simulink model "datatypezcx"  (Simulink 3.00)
settings: Solver=FixedStepDiscrete  SolverMode=SingleTasking  StartTime=0.0  StopTime=4  FixedStep=.01  RelTol=1e-3

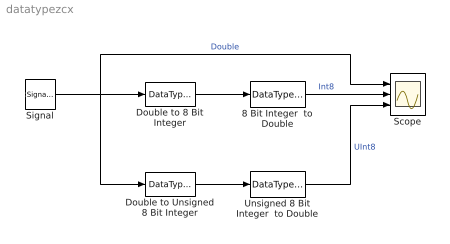
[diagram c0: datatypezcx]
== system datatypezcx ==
  8 Bit Integer  to Double : DataTypeConversion  DataType=double  SaturateOnIntegerOverflow=on
  Double to 8 Bit Integer : DataTypeConversion  DataType=int8  SaturateOnIntegerOverflow=on
  Double to Unsigned 8 Bit Integer : DataTypeConversion  DataType=uint8  SaturateOnIntegerOverflow=on
  Scope : Scope  NumInputPorts=3
  Signal : SignalGenerator  WaveForm=sine  Amplitude=150  Frequency=1  Units=Hertz
  Unsigned 8 Bit Integer  to Double : DataTypeConversion  DataType=double  SaturateOnIntegerOverflow=on
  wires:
  Double to 8 Bit Integer/1 -> 8 Bit Integer  to Double/1
  8 Bit Integer  to Double/1 -> Scope/2  "Int8"
  Signal/1 -> Double to 8 Bit Integer/1, Scope/1, Double to Unsigned 8 Bit Integer/1  "Double"
  Unsigned 8 Bit Integer  to Double/1 -> Scope/3  "UInt8"
  Double to Unsigned 8 Bit Integer/1 -> Unsigned 8 Bit Integer  to Double/1
